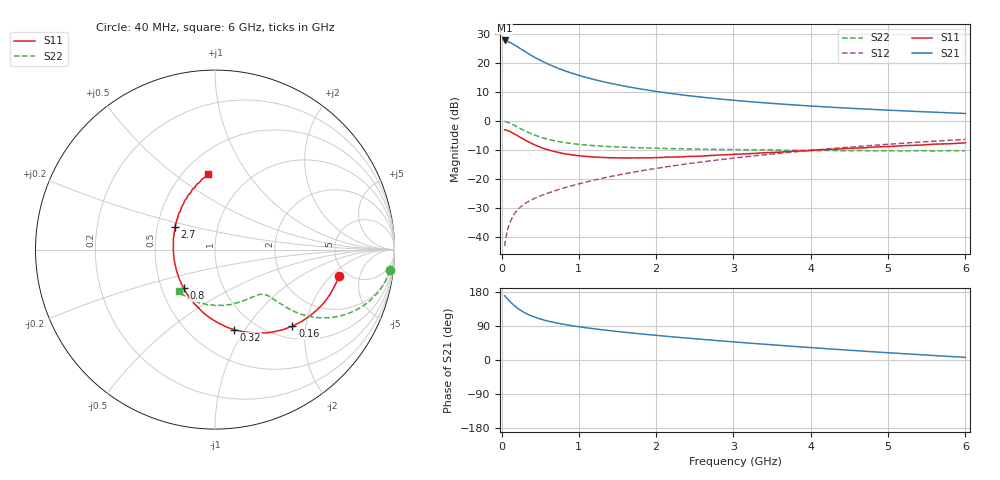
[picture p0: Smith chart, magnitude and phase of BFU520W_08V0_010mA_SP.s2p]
! Filename:  P:\Prog\Test\Noise\ATS_data\Testdata_Net\Run2\BFU520W_APM2013_06_A05_08p0V_010mA_SP_CM01_D.s2p
! Date/Time: Tue 26/Mar/2013 18:01:42
! BFU520W_APM2013_06_A05_08p0V_1to20mA_SP_CM01_Bias6_R.s2p
! MDIF S-parameter v. bias file
! BFU520W_APM2013_06_A05_08p0V_1to20mA_SP_CM01
! Date/time Thu Mar 21 15:28:29 2013
! VAR V_out= 8.0000
! VAR I_out= 10.0050
! VAR V_in= 0.8267
! VAR I_in= 0.1094
! Device data file deembeded for feedlines and parallel
! Original file: \Run2\BFU520W_APM2013_06_A05_08p0V_010mA_SP_CM01_R.s2p
! Feed-files: PR019V01_070313_Feed1.s2p, PR019V01_070313_Feed2.s2p
! Parallel-file: PR019V01_070313_Par.s2p
# MHz S MA R 50
!  Freq-MHz  S11-mag  S11-arg  S21-mag  S21-arg  S12-mag  S12-arg  S22-mag  S22-arg
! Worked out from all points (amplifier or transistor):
!   98 points, 40 MHz to 6 GHz, reference 50 ohm
!   highest |S21| = 27.7 dB at 40 MHz (marker M1)
!   |S21| within 3 dB of that: start of sweep to 256.2 MHz
!   unconditionally stable (mu >= 1): 1.479 GHz to 2.667 GHz
!   at 300 MHz: K = 0.51, MSG = 26.2 dB, |S12| = -28.4 dB
!   at 1.6 GHz: K = 1.01, MAG = 14.5 dB, |S12| = -18.1 dB
!   at 6 GHz: K = 0.88, MSG = 4.5 dB, |S12| = -6.3 dB
!   S11 on the Smith chart (normalised r, x): 40 MHz: 4.27, -2.48; 160 MHz: 1.25, -1.69; 320 MHz: 0.79, -0.89; 800 MHz: 0.65, -0.30; 2.7 GHz: 0.62, +0.16; 6 GHz: 0.66, +0.67
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40  0.7047 -12.0  24.13 169.7  0.007085 84.1  0.9807 -6.8
50  0.7011 -14.9  24.09 167.3  0.008766 82.9  0.9752 -8.4
60  0.6947 -17.9  23.59 164.9  0.01041 81.4  0.9672 -10.2
80  0.6814 -23.7  23.16 160.5  0.01363 78.8  0.9489 -13.3
100  0.665 -29.2  22.5 156.2  0.01666 76.6  0.9262 -16.2
120  0.6459 -34.7  21.95 152.0  0.01949 74.5  0.9026 -18.9
160  0.6068 -44.7  20.46 144.6  0.02468 70.8  0.8503 -23.6
220  0.546 -58.1  18.34 134.9  0.03102 67.1  0.7709 -29.0
280  0.4906 -69.5  16.29 127.1  0.03629 64.7  0.7002 -32.9
320  0.4581 -76.5  15.11 122.6  0.0394 63.8  0.6594 -34.7
400  0.4051 -88.3  13.04 115.4  0.04496 62.9  0.5919 -37.0
500  0.356 -101.0  11.03 108.4  0.05142 62.8  0.5299 -38.7
650  0.3065 -116.3  8.903 100.4  0.06084 63.6  0.4681 -39.6
800  0.2763 -129.2  7.425 94.3  0.07035 64.6  0.4297 -40.3
1050  0.2495 -146.5  5.81 86.3  0.08667 66.0  0.391 -41.1
1500  0.2326 -170.2  4.184 75.2  0.1175 66.8  0.3579 -44.2
2050  0.2356 169.1  3.146 64.1  0.157 66.0  0.3395 -50.2
2700  0.2552 150.9  2.474 52.7  0.206 63.4  0.3268 -60.1
3100  0.2711 141.2  2.207 46.3  0.2379 61.3  0.3219 -66.5
4100  0.3183 122.5  1.776 31.3  0.321 54.5  0.311 -86.1
5200  0.377 105.7  1.491 16.6  0.4155 45.3  0.306 -110.7
6000  0.4213 95.1  1.345 7.1  0.4823 37.7  0.3074 -130.9
